| TEXAS INSTRUMENTS INCORPORATED
| Standard Linear and Logic Group
| IBIS Model of SN74AHC240
| OCTAL BUFFERS/DRIVERS WITH 3-STATE OUTPUTS
| This file contains package information for the following:
|  PDIP 20-pin (N) package as [Component] AHC240_N
|  SOIC 20-pin (DW) package as [Component] AHC240_DW
|  SOP 20-pin (NS) package as [Component] AHC240_NS
|  SSOP 20-pin (DB) package as [Component] AHC240_DB
|  TSSOP 20-pin (PW) package as [Component] AHC240_PW
|  TVSOP 20-pin (DGV) package as [Component] AHC240_DGV
| This device can be powered at the following Vccs:
|  5 volt Vcc
|  3.3 volt Vcc
| This file provides unique models under the [Model Selector] for each Vcc.
| For operation at a specific Vcc, select the appropriate model after each
| [Model Selector] keyword.
[IBIS Ver]   3.2
[Comment char]  |_char
[File Name]   sn74ahc240.ibs
[File Rev]   1.1 | a_die
[Date]   April 28, 2006
[Source]   Data created from TI-SPICE simulations at TI-SLL.
[Notes]   The following is an IBIS list for the SN74AHC240.
   Please contact sllibis@ti.com with questions and
   comments concerning SLL IBIS models.
   This IBIS model is created from a BA (back annotated netlist)
   - FILE REV HISTORY
   - 1.1 Release IBIS file on 05/09/06
   - C_comp values are taken at a different test condition
   than the data sheet.
   - Power clamp data deleted as there is no power-clamp diode.
[Disclaimer] Property of Texas Instruments Incorporated.  Unauthorized
   reproduction and/or distribution is strictly prohibited.
   This product is protected under copyright law.
   Created  2006, (C) Copyright  2006, Texas Instruments
   Incorporated, All Rights Reserved
   UNLESS THERE IS A SIGNED, WRITTEN AGREEMENT TO THE
   CONTRARY, TEXAS INSTRUMENTS (TI) IS PROVIDING THE IBIS
   MODELS  AND WITHOUT ANY WARRANTY, EXPRESSED OR
   IMPLIED.  TI assumes no liability for:
   1) the accuracy of the IBIS models provided to your
   company;
   2) the proper functioning of these IBIS Models in your
   design or for any resulting applications; or
   3) infringement of patents, copyrights or intellectual
   property rights resulting from your use of these IBIS
   models.
   TI provides IBIS Models as a service to our customers.
   You and your company shall not distribute, sell or give
   these models to anyone else without prior written
   permission from TI.
   TI reserves the right to make changes to our products or
   to discontinue any semiconductor product or service
   without notice, and advises our customers to obtain the
   latest version of relevant information to verify, before
   placing orders, that the information being relied on is
   current.
   Please be aware that your receipt and use of the IBIS
   information provided shall serve as acceptance of these
   terms and conditions.  If you do not accept these terms,
   you should return or destroy the IBIS models and any
   other accompanying information immediately.
| Component SN74AHC240_N 20-PIN PDIP
[Component]   SN74AHC240_N
[Manufacturer]   Texas Instruments, Inc.
[Package]
|   typ   min   max
R_pkg   4.300e-02   3.800e-02   5.000e-02
L_pkg   7.384e-09   4.680e-09   1.032e-08
C_pkg   5.100e-13   2.310e-13   8.210e-13
[Pin]   signal_name   model_name   R_pin   L_pin   C_pin
1   N1OE   AHC240_NOE   4.200e-02   9.427e-09   8.100e-13
2   1A1   AHC240_IN   4.600e-02   8.544e-09   4.560e-13
3   2Y4   AHC240_IO   4.800e-02   7.163e-09   4.350e-13
4   1A2   AHC240_IN   4.000e-02   4.825e-09   2.610e-13
5   2Y3   AHC240_IO   4.000e-02   5.284e-09   6.480e-13
6   1A3   AHC240_IN   4.000e-02   4.686e-09   2.320e-13
7   2Y2   AHC240_IO   4.000e-02   6.359e-09   4.890e-13
8   1A4   AHC240_IN   3.800e-02   7.982e-09   4.750e-13
9   2Y1   AHC240_IO   4.300e-02   9.403e-09   4.750e-13
10   GND   GND   5.000e-02   1.032e-08   8.050e-13
11   2A1   AHC240_IN   5.000e-02   1.028e-08   8.100e-13
12   1Y4   AHC240_IO   4.300e-02   9.383e-09   4.770e-13
13   2A2   AHC240_IN   3.800e-02   7.978e-09   4.760e-13
14   1Y3   AHC240_IO   4.000e-02   6.302e-09   4.920e-13
15   2A3   AHC240_IN   4.000e-02   4.680e-09   2.310e-13
16   1Y2   AHC240_IO   4.000e-02   5.284e-09   6.480e-13
17   2A4   AHC240_IN   4.000e-02   4.822e-09   2.610e-13
18   1Y1   AHC240_IO   4.700e-02   7.118e-09   4.390e-13
19   N2OE   AHC240_NOE   4.600e-02   8.492e-09   4.610e-13
20   VCC   POWER   4.300e-02   9.348e-09   8.210e-13
| Component SN74AHC240_DW 20-PIN SOIC
[Component]   SN74AHC240_DW
[Manufacturer]   Texas Instruments, Inc.
[Package]
|   typ   min   max
R_pkg   3.800e-02   3.300e-02   4.500e-02
L_pkg   5.012e-09   4.110e-09   6.349e-09
C_pkg   7.170e-13   5.300e-13   8.680e-13
[Pin]   signal_name   model_name   R_pin   L_pin   C_pin
1   N1OE   AHC240_NOE   4.200e-02   6.336e-09   8.650e-13
2   1A1   AHC240_IN   4.300e-02   5.542e-09   8.670e-13
3   2Y4   AHC240_IO   3.400e-02   4.714e-09   7.320e-13
4   1A2   AHC240_IN   3.400e-02   4.377e-09   5.910e-13
5   2Y3   AHC240_IO   3.600e-02   4.130e-09   5.330e-13
6   1A3   AHC240_IN   3.500e-02   4.111e-09   5.300e-13
7   2Y2   AHC240_IO   3.400e-02   4.284e-09   5.830e-13
8   1A4   AHC240_IN   3.400e-02   4.634e-09   7.260e-13
9   2Y1   AHC240_IO   4.000e-02   5.518e-09   8.650e-13
10   GND   GND   4.300e-02   6.349e-09   8.660e-13
11   2A1   AHC240_IN   4.100e-02   6.281e-09   8.610e-13
12   1Y4   AHC240_IO   4.500e-02   5.561e-09   8.680e-13
13   2A2   AHC240_IN   3.300e-02   4.778e-09   7.420e-13
14   1Y3   AHC240_IO   3.500e-02   4.414e-09   5.960e-13
15   2A3   AHC240_IN   3.500e-02   4.110e-09   5.330e-13
16   1Y2   AHC240_IO   3.600e-02   4.130e-09   5.330e-13
17   2A4   AHC240_IN   3.400e-02   4.377e-09   5.910e-13
18   1Y1   AHC240_IO   3.400e-02   4.714e-09   7.310e-13
19   N2OE   AHC240_NOE   4.300e-02   5.569e-09   8.680e-13
20   VCC   POWER   4.200e-02   6.308e-09   8.640e-13
| Component SN74AHC240_NS 20-PIN SOP
[Component]   SN74AHC240_NS
[Manufacturer]   Texas Instruments, Inc.
[Package]
|   typ   min   max
R_pkg   4.400e-02   2.900e-02   5.800e-02
L_pkg   3.666e-09   2.317e-09   5.115e-09
C_pkg   5.480e-13   3.160e-13   7.250e-13
[Pin]   signal_name   model_name   R_pin   L_pin   C_pin
1   N1OE   AHC240_NOE   5.800e-02   5.115e-09   7.250e-13
2   1A1   AHC240_IN   5.300e-02   4.591e-09   7.240e-13
3   2Y4   AHC240_IO   4.900e-02   3.754e-09   5.720e-13
4   1A2   AHC240_IN   2.900e-02   2.549e-09   3.880e-13
5   2Y3   AHC240_IO   3.100e-02   2.317e-09   3.160e-13
6   1A3   AHC240_IN   3.100e-02   2.317e-09   3.160e-13
7   2Y2   AHC240_IO   2.900e-02   2.556e-09   3.990e-13
8   1A4   AHC240_IN   4.900e-02   3.754e-09   5.790e-13
9   2Y1   AHC240_IO   5.300e-02   4.591e-09   7.240e-13
10   GND   GND   5.800e-02   5.115e-09   7.250e-13
11   2A1   AHC240_IN   5.800e-02   5.115e-09   7.250e-13
12   1Y4   AHC240_IO   5.300e-02   4.591e-09   7.240e-13
13   2A2   AHC240_IN   4.900e-02   3.754e-09   5.790e-13
14   1Y3   AHC240_IO   2.900e-02   2.557e-09   3.990e-13
15   2A3   AHC240_IN   3.100e-02   2.317e-09   3.160e-13
16   1Y2   AHC240_IO   3.100e-02   2.317e-09   3.160e-13
17   2A4   AHC240_IN   2.900e-02   2.557e-09   3.990e-13
18   1Y1   AHC240_IO   4.900e-02   3.754e-09   5.790e-13
19   N2OE   AHC240_NOE   5.300e-02   4.591e-09   7.240e-13
20   VCC   POWER   5.800e-02   5.115e-09   7.250e-13
| Component SN74AHC240_DB 20-PIN SSOP
[Component]   SN74AHC240_DB
[Manufacturer]   Texas Instruments, Inc.
[Package]
|   typ   min   max
R_pkg   4.000e-02   3.500e-02   5.100e-02
L_pkg   3.495e-09   3.035e-09   4.314e-09
C_pkg   4.200e-13   3.460e-13   5.020e-13
[Pin]   signal_name   model_name   R_pin   L_pin   C_pin
1   N1OE   AHC240_NOE   4.900e-02   4.310e-09   5.020e-13
2   1A1   AHC240_IN   4.800e-02   3.903e-09   4.870e-13
3   2Y4   AHC240_IO   3.500e-02   3.189e-09   3.960e-13
4   1A2   AHC240_IN   3.500e-02   3.036e-09   3.470e-13
5   2Y3   AHC240_IO   3.500e-02   3.035e-09   3.670e-13
6   1A3   AHC240_IN   3.500e-02   3.035e-09   3.670e-13
7   2Y2   AHC240_IO   3.500e-02   3.036e-09   3.470e-13
8   1A4   AHC240_IN   3.500e-02   3.189e-09   3.970e-13
9   2Y1   AHC240_IO   4.700e-02   3.899e-09   4.880e-13
10   GND   GND   5.100e-02   4.314e-09   5.000e-13
11   2A1   AHC240_IN   5.100e-02   4.314e-09   5.000e-13
12   1Y4   AHC240_IO   4.700e-02   3.899e-09   4.880e-13
13   2A2   AHC240_IN   3.500e-02   3.189e-09   3.970e-13
14   1Y3   AHC240_IO   3.500e-02   3.036e-09   3.460e-13
15   2A3   AHC240_IN   3.500e-02   3.035e-09   3.670e-13
16   1Y2   AHC240_IO   3.500e-02   3.035e-09   3.670e-13
17   2A4   AHC240_IN   3.500e-02   3.036e-09   3.460e-13
18   1Y1   AHC240_IO   3.500e-02   3.189e-09   3.970e-13
19   N2OE   AHC240_NOE   4.700e-02   3.899e-09   4.880e-13
20   VCC   POWER   5.100e-02   4.314e-09   5.020e-13
| Component SN74AHC240_PW 20-PIN TSSOP
[Component]   SN74AHC240_PW
[Manufacturer]   Texas Instruments, Inc.
[Package]
|   typ   min   max
R_pkg   5.000e-02   4.200e-02   6.000e-02
L_pkg   2.802e-09   2.248e-09   3.553e-09
C_pkg   3.170e-13   2.020e-13   4.430e-13
[Pin]   signal_name   model_name   R_pin   L_pin   C_pin
1   N1OE   AHC240_NOE   5.500e-02   3.461e-09   4.400e-13
2   1A1   AHC240_IN   5.500e-02   3.150e-09   4.010e-13
3   2Y4   AHC240_IO   4.200e-02   2.619e-09   3.020e-13
4   1A2   AHC240_IN   4.500e-02   2.273e-09   2.020e-13
5   2Y3   AHC240_IO   4.500e-02   2.248e-09   2.240e-13
6   1A3   AHC240_IN   4.500e-02   2.273e-09   2.260e-13
7   2Y2   AHC240_IO   4.400e-02   2.323e-09   2.050e-13
8   1A4   AHC240_IN   4.600e-02   2.704e-09   3.070e-13
9   2Y1   AHC240_IO   6.000e-02   3.265e-09   4.110e-13
10   GND   GND   5.700e-02   3.506e-09   4.360e-13
11   2A1   AHC240_IN   5.800e-02   3.553e-09   4.370e-13
12   1Y4   AHC240_IO   5.800e-02   3.193e-09   4.050e-13
13   2A2   AHC240_IN   4.200e-02   2.704e-09   3.110e-13
14   1Y3   AHC240_IO   4.600e-02   2.392e-09   2.100e-13
15   2A3   AHC240_IN   4.700e-02   2.334e-09   2.290e-13
16   1Y2   AHC240_IO   4.700e-02   2.300e-09   2.270e-13
17   2A4   AHC240_IN   4.700e-02   2.349e-09   2.070e-13
18   1Y1   AHC240_IO   4.500e-02   2.677e-09   3.060e-13
19   N2OE   AHC240_NOE   6.000e-02   3.235e-09   4.060e-13
20   VCC   POWER   5.600e-02   3.487e-09   4.430e-13
| Component SN74AHC240_DGV 20-PIN TVSOP
[Component]   SN74AHC240_DGV
[Manufacturer]   Texas Instruments, Inc.
[Package]
|   typ   min   max
R_pkg   4.400e-02   3.800e-02   4.800e-02
L_pkg   2.561e-09   2.236e-09   2.961e-09
C_pkg   3.420e-13   2.640e-13   4.460e-13
[Pin]   signal_name   model_name   R_pin   L_pin   C_pin
1   N1OE   AHC240_NOE   4.400e-02   2.935e-09   4.170e-13
2   1A1   AHC240_IN   4.200e-02   2.869e-09   4.460e-13
3   2Y4   AHC240_IO   4.300e-02   2.399e-09   3.160e-13
4   1A2   AHC240_IN   4.400e-02   2.236e-09   2.650e-13
5   2Y3   AHC240_IO   4.600e-02   2.278e-09   2.640e-13
6   1A3   AHC240_IN   4.500e-02   2.274e-09   2.640e-13
7   2Y2   AHC240_IO   4.400e-02   2.285e-09   2.690e-13
8   1A4   AHC240_IN   4.300e-02   2.452e-09   3.200e-13
9   2Y1   AHC240_IO   4.400e-02   2.900e-09   4.460e-13
10   GND   GND   4.400e-02   2.961e-09   4.180e-13
11   2A1   AHC240_IN   4.500e-02   2.954e-09   4.180e-13
12   1Y4   AHC240_IO   4.200e-02   2.847e-09   4.430e-13
13   2A2   AHC240_IN   4.500e-02   2.453e-09   3.190e-13
14   1Y3   AHC240_IO   4.500e-02   2.297e-09   2.690e-13
15   2A3   AHC240_IN   4.800e-02   2.334e-09   2.680e-13
16   1Y2   AHC240_IO   4.800e-02   2.335e-09   2.670e-13
17   2A4   AHC240_IN   4.600e-02   2.299e-09   2.680e-13
18   1Y1   AHC240_IO   4.600e-02   2.457e-09   3.200e-13
19   N2OE   AHC240_NOE   4.300e-02   2.848e-09   4.410e-13
20   VCC   POWER   3.800e-02   2.812e-09   4.080e-13
| Model AHC240_NOE
[Model Selector]   AHC240_NOE
AHC240_NOE_50   5 volt Vcc
AHC240_NOE_33   3.3 volt Vcc
| Model AHC240_IN
[Model Selector]   AHC240_IN
AHC240_IN_50   5 volt Vcc
AHC240_IN_33   3.3 volt Vcc
| Model AHC240_IO
[Model Selector]   AHC240_IO
AHC240_IO_50   5 volt Vcc
AHC240_IO_33   3.3 volt Vcc
| Models and submodels in the file (6): AHC240_NOE_50 (Input), AHC240_NOE_33 (Input), AHC240_IN_50 (Input), AHC240_IN_33 (Input), AHC240_IO_50 (3-state), AHC240_IO_33 (3-state)
